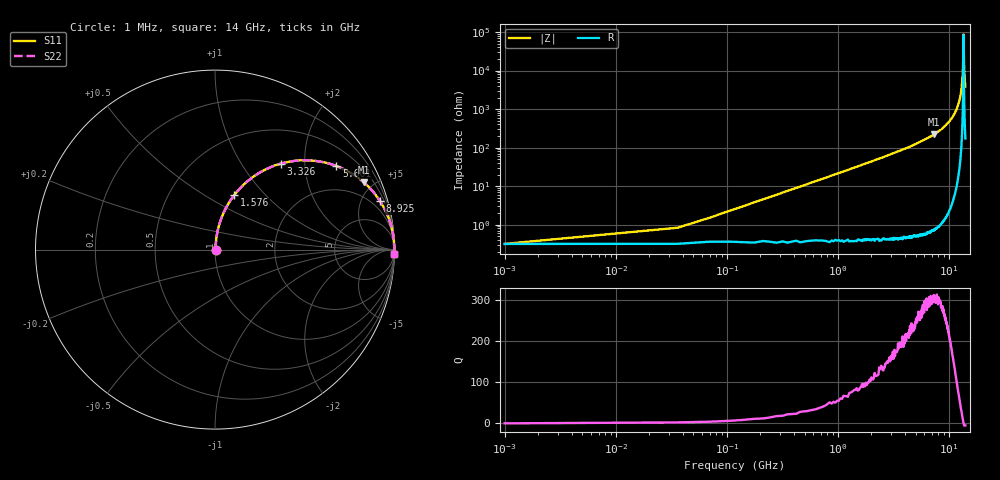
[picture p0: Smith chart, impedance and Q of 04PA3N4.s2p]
! Coilcraft 0402PA-3N4 Chip Inductor
! 11 March 2004
# MHZ S MA R 50
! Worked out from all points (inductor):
!   401 points, 1 MHz to 14 GHz, reference 50 ohm
!   read as one part in series: L = 3.39 nH near 71 MHz
!   highest Q = 305 at 7.315 GHz (marker M1), where L = 4.82 nH
!   self-resonance near 13.48 GHz
!   S11 on the Smith chart (normalised r, x): 1 MHz: 1.01, +0.00; 1.576 GHz: 1.01, +0.68; 3.326 GHz: 1.01, +1.51; 5.601 GHz: 1.01, +2.89; 8.925 GHz: 1.03, +6.79; 14 GHz: 6, -76
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1  0.003312 3.7  0.997 -0.0  0.997 -0.0  0.003312 3.7
175.987  0.038 82.5  0.996 -2.1  0.996 -2.1  0.038 82.5
385.972  0.082 82.8  0.993 -4.7  0.993 -4.7  0.082 82.8
840.94  0.177 78.6  0.981 -10.2  0.981 -10.2  0.177 78.6
1575.887  0.322 70.6  0.943 -18.8  0.943 -18.8  0.322 70.6
2345.832  0.458 62.3  0.886 -27.2  0.886 -27.2  0.458 62.3
3325.762  0.602 52.7  0.795 -37.0  0.795 -37.0  0.602 52.7
4690.665  0.75 41.1  0.658 -48.6  0.658 -48.6  0.75 41.1
5600.6  0.821 34.6  0.568 -55.2  0.568 -55.2  0.821 34.6
7000.5  0.897 26.0  0.438 -63.8  0.438 -63.8  0.897 26.0
7315.478  0.91 24.3  0.411 -65.5  0.411 -65.5  0.91 24.3
8925.363  0.958 16.4  0.282 -73.4  0.282 -73.4  0.958 16.4
9345.333  0.967 14.6  0.252 -75.2  0.252 -75.2  0.967 14.6
11690.17  0.994 5.7  0.099 -83.8  0.099 -83.8  0.994 5.7
12495.11  0.998 3.0  0.053 -85.9  0.053 -85.9  0.998 3.0
12950.08  0.999 1.6  0.028 -86.2  0.028 -86.2  0.999 1.6
13265.05  0.999 0.6  0.011 -83.7  0.011 -83.7  0.999 0.6
13475.04  0.999 0.0  0.001153 -12.8  0.001153 -12.8  0.999 0.0
13545.03  0.999 -0.2  0.003525 71.1  0.003525 71.1  0.999 -0.2
13615.03  0.999 -0.4  0.007007 80.2  0.007007 80.2  0.999 -0.4
13720.02  0.999 -0.7  0.012 83.9  0.012 83.9  0.999 -0.7
14000  0.998 -1.5  0.026 85.9  0.026 85.9  0.998 -1.5
